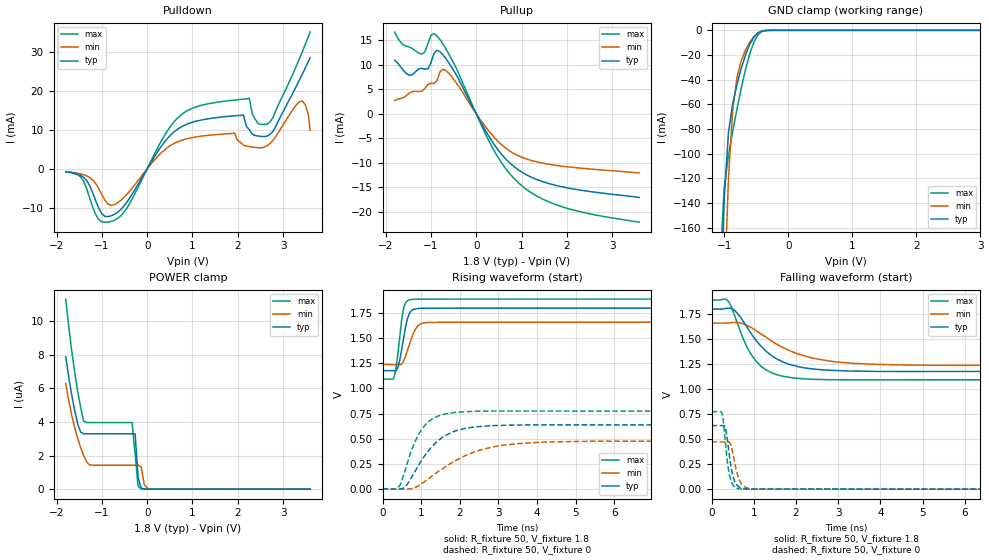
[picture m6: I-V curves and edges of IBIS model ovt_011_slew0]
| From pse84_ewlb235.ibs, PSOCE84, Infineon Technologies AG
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[Model] ovt_011_slew0
Model_type I/O
Enable   Active-High
Vinl  =  0.54
Vinh  =  1.26
Vmeas =  0.9
Cref  =  15e-12
| Capacitance   typ   min   max
C_comp   1.39974e-12   1.35992e-12   1.44753e-12
| Variables   typ   min   max
[GND Clamp Reference]   0   0   0
[POWER Clamp Reference]   1.8   1.66   1.89
[Pulldown Reference]   0   0   0
[Pullup Reference]   1.8   1.66   1.89
[Temperature Range]   25   125   -40
[Voltage Range]   1.8   1.66   1.89
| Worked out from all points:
|   slope of the pulldown table from 0 to 0.27 V, typ, clamps not added: 53.3 ohm
|   slope of the pullup table from 0 to 0.27 V, typ, clamps not added: 60.8 ohm
|   GND clamp passes 1 mA (typ) near -0.43 V on its own axis
|   falling waveform, R_fixture 50, V_fixture 1.8: 20-80 % time 794ps typ, 1.19ns min, 564ps max; typ from 1.8 V to 1.18 V
|   falling waveform, R_fixture 50, V_fixture 0: 20-80 % time 138ps typ, 160ps min, 123ps max; typ from 0.636 V to 0 V
|   rising waveform, R_fixture 50, V_fixture 1.8: 20-80 % time 178ps typ, 236ps min, 147ps max; typ from 1.18 V to 1.8 V
|   rising waveform, R_fixture 50, V_fixture 0: 20-80 % time 768ps typ, 1.3ns min, 509ps max; typ from 0 V to 0.636 V
[GND Clamp]
| Voltage   I(typ)   I(min)   I(max)
-1.271V   -717.5mA   -832.8mA   -643.6mA
-1.07V    -241.9mA   -348.3mA   -192.2mA
-1.003V   -137.2mA   -218.1mA   -128.1mA
-936.6mV  -83.06mA   -120.7mA   -101.3mA
-869.7mV  -59.26mA   -64.32mA   -81.77mA
-802.8mV  -43.7mA    -38.08mA   -63.69mA
-735.9mV  -30.76mA   -24.63mA   -46.83mA
-602.1mV  -11.27mA   -9.362mA   -18.72mA
-535.2mV  -5.241mA   -4.803mA   -9.042mA
-468.3mV  -1.746mA   -1.965mA   -3.086mA
-334.5mV  -35.9uA    -120.8uA   -33.39uA
3.6V      0A         0A         0A
[POWER Clamp]
| Voltage   I(typ)   I(min)   I(max)
-1.8V     7.872uA    6.273uA    11.31uA
-1.672V   5.671uA    4.461uA    8.32uA
-1.539V   3.91uA     3.037uA    5.87uA
-1.405V   3.295uA    2.008uA    4.063uA
-1.271V   3.295uA    1.447uA    3.964uA
-334.5mV  3.295uA    1.429uA    3.964uA
-267.6mV  3.295uA    1.429uA    2.099uA
-200.7mV  664.1nA    1.429uA    166.6nA
-133.8mV  69.92nA    1.319uA    14.86nA
-66.9mV   7.33nA     291.5nA    4.066nA
62.07mV   0A         0A         0A
3.6V      0A         0A         0A
[Pulldown]
| Voltage   I(typ)   I(min)   I(max)
-1.8V     -821.3uA   -770uA     -752.7uA
-1.405V   -2.23mA    -1.552mA   -3.186mA
-1.07V    -10.15mA   -5.122mA   -13.1mA
-669mV    -11.29mA   -8.877mA   -12.89mA
806.9mV   11.06mA    7.464mA    14.33mA
2.126V    13.78mA    6.047mA    17.85mA
2.256V    10.01mA    5.677mA    18.03mA
2.452V    8.367mA    5.375mA    11.54mA
2.712V    8.833mA    6.447mA    11.99mA
3.364V    22.79mA    17.19mA    28.26mA
3.494V    25.92mA    16.43mA    31.95mA
3.6V      28.52mA    9.831mA    35.06mA
[Pullup]
| Voltage   I(typ)   I(min)   I(max)
-1.8V     10.97mA    2.706mA    16.69mA
-1.672V   9.603mA    3.116mA    14.62mA
-1.472V   7.853mA    4.268mA    13.62mA
-1.204V   9.253mA    4.613mA    12.18mA
-1.07V    9.157mA    5.942mA    14.22mA
-936.6mV  12.25mA    6.16mA     16.37mA
-735.9mV  12.06mA    9.113mA    14.26mA
-535.2mV  9.366mA    7.503mA    10.99mA
372.4mV   -5.939mA   -4.563mA   -7.158mA
1.055V    -12.19mA   -9.054mA   -15.06mA
1.996V    -15.1mA    -10.81mA   -19.27mA
3.6V      -17.08mA   -12.08mA   -22.15mA
[Ramp]
dV/dt_r   0.381715/0.767812n  0.283782/1.30386n  0.464622/0.509257n
dV/dt_f   0.373486/0.793793n  0.252676/1.18884n  0.47771/0.564016n
R_load = 50
[Falling Waveform]
R_fixture = 50
V_fixture = 1.8
V_fixture_min = 1.66
V_fixture_max = 1.89
| Time   V(typ)   V(min)   V(max)
0s        1.8V       1.66V      1.89V
393.4ps   1.81V      1.661V     1.88V
586.5ps   1.77V      1.667V     1.689V
843.5ps   1.617V     1.637V     1.418V
1.051ns   1.49V      1.586V     1.282V
1.25ns    1.396V     1.529V     1.203V
1.667ns   1.276V     1.421V     1.131V
2.037ns   1.226V     1.354V     1.109V
3.219ns   1.182V     1.263V     1.093V
800ns     1.178V     1.239V     1.094V
[Falling Waveform]
R_fixture = 50
V_fixture = 0
V_fixture_min = 0
V_fixture_max = 0
| Time   V(typ)   V(min)   V(max)
0s        636.2mV    473mV      774.4mV
248.5ps   636mV      473mV      755.6mV
281.7ps   637mV      473mV      669.1mV
336.3ps   595.8mV    472.8mV    427.6mV
400.7ps   406.2mV    473.4mV    193.4mV
477.5ps   182.3mV    408.9mV    64.74mV
548.4ps   78.2mV     263.4mV    21.08mV
642.1ps   24.15mV    107.3mV    3.873mV
796.3ps   3.248mV    21.28mV    613.8uV
800ns     25.74nV    1.294uV    12.09nV
[Rising Waveform]
R_fixture = 50
V_fixture = 1.8
V_fixture_min = 1.66
V_fixture_max = 1.89
| Time   V(typ)   V(min)   V(max)
0s        1.178V     1.239V     1.094V
303.3ps   1.178V     1.239V     1.12V
358.2ps   1.18V      1.239V     1.227V
420.9ps   1.242V     1.239V     1.428V
527.7ps   1.46V      1.26V      1.762V
617.1ps   1.649V     1.346V     1.863V
726.1ps   1.765V     1.473V     1.885V
928.5ps   1.797V     1.628V     1.889V
1.489ns   1.799V     1.659V     1.89V
800ns     1.8V       1.66V      1.89V
[Rising Waveform]
R_fixture = 50
V_fixture = 0
V_fixture_min = 0
V_fixture_max = 0
| Time   V(typ)   V(min)   V(max)
0s        25.74nV    1.294uV    12.09nV
434.3ps   -2.314mV   -153.7uV   27.85mV
620.4ps   35.67mV    -1.793mV   234.2mV
913.2ps   223.2mV    26.87mV    527.6mV
1.247ns   405.7mV    118.2mV    685.5mV
1.816ns   567.2mV    264.7mV    757.4mV
2.721ns   626.7mV    404.8mV    774.8mV
4.154ns   637.4mV    465.7mV    774.6mV
6.273ns   636.5mV    474.7mV    774.3mV
800ns     636.2mV    473mV      774.4mV
